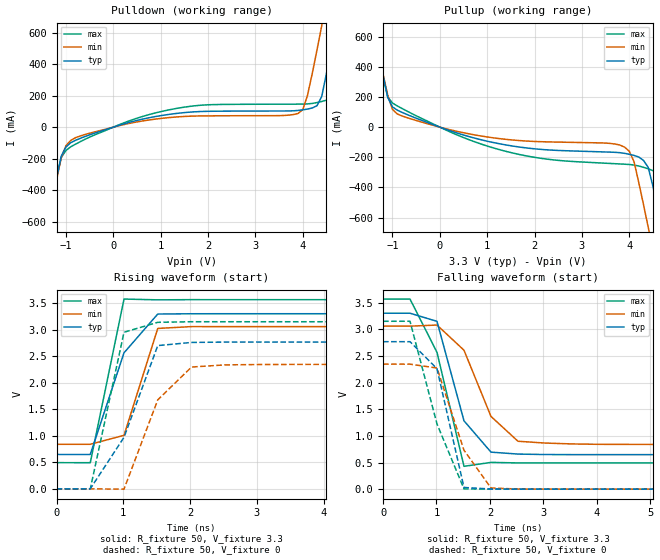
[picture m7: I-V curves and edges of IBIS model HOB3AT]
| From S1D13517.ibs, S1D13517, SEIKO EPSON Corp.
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[Model]   HOB3AT
Model_type Output
Polarity Non-Inverting
C_comp   5p   4p   6p
[Temperature Range] 50   100   0
[Voltage Range]   3.3   3.0   3.6
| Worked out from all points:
|   slope of the pulldown table from 0 to 0.495 V, typ, clamps not added: 11.6 ohm
|   slope of the pullup table from 0 to 0.495 V, typ, clamps not added: 9.57 ohm
|   falling waveform, R_fixture 50, V_fixture 3.3: 20-80 % time 492ps typ, 602ps min, 539ps max; typ from 3.3 V to 0.648 V
|   falling waveform, R_fixture 50, V_fixture 0: 20-80 % time 376ps typ, 562ps min, 586ps max; typ from 2.77 V to 0 V
|   rising waveform, R_fixture 50, V_fixture 3.3: 20-80 % time 508ps typ, 334ps min, 302ps max; typ from 0.648 V to 3.3 V
|   rising waveform, R_fixture 50, V_fixture 0: 20-80 % time 580ps typ, 525ps min, 323ps max; typ from 0 V to 2.77 V
[Pullup]
-3.3V     3.943A     3.608A     4.348A
-1.4V     684.1mA    660.3mA    712.3mA
-1.1V     197.5mA    211.2mA    200.1mA
-800mV    98.34mA    74.29mA    124mA
1.4V      -118.4mA   -81.14mA   -161mA
3.9V      -173.8mA   -132.3mA   -245.9mA
4.1V      -187.6mA   -228.8mA   -251.3mA
4.4V      -266.9mA   -664.2mA   -276.6mA
4.7V      -721.9mA   -1.12A     -342.9mA
4.9V      -1.059A    -1.425A    -612.4mA
5V        -1.228A    -1.577A    -799.5mA
6.6V      -3.945A    -4.028A    -3.853A
[Pulldown]
-3.3V     -3.888A    -3.547A    -4.327A
-1.4V     -659.3mA   -637.4mA   -695.5mA
-1.1V     -183.5mA   -194.3mA   -193.3mA
-1V       -126mA     -116.8mA   -148.1mA
-700mV    -71.52mA   -56.26mA   -92.68mA
1.4V      89.34mA    66.11mA    122.4mA
3.9V      106.1mA    86.91mA    146.2mA
4.1V      114.9mA    202.9mA    147.6mA
4.4V      194.9mA    644.6mA    163.1mA
4.7V      675.1mA    1.105A     215.6mA
5V        1.186A     1.566A     718.4mA
6.6V      3.921A     4.037A     3.78A
[Falling Waveform]
R_fixture=50
V_fixture=3.3
0s        3.3V       3.057V     3.565V
505.1ps   3.3V       3.057V     3.566V
1.01ns    3.148V     3.078V     2.567V
1.515ns   1.282V     2.606V     428.5mV
2.02ns    694.6mV    1.364V     502.2mV
2.525ns   658mV      898.6mV    492.3mV
3.03ns    649.5mV    864.9mV    493.1mV
4.04ns    647.6mV    840.8mV    493mV
5.051ns   647.6mV    838.9mV    492.9mV
50ns      647.6mV    838.8mV    492.9mV
[Falling Waveform]
R_fixture=50
V_fixture=0
0s        2.766V     2.344V     3.149V
505.1ps   2.766V     2.344V     3.149V
1.01ns    2.259V     2.272V     1.223V
1.515ns   31.88mV    730.2mV    4.675mV
2.02ns    2.635mV    23.03mV    803.6uV
2.525ns   682.4uV    2.289mV    177uV
50ns      13.34uV    657.6nV    1.085uV
[Rising Waveform]
R_fixture=50
V_fixture=3.3
0s        647.6mV    838.8mV    492.9mV
505.1ps   647.7mV    838.9mV    491.8mV
1.01ns    2.564V     1.008V     3.576V
1.515ns   3.294V     3.023V     3.562V
2.02ns    3.299V     3.057V     3.565V
50ns      3.3V       3.057V     3.565V
[Rising Waveform]
R_fixture=50
V_fixture=0
0s        0V         0V         0V
505.1ps   11.85uV    -10.88uV   -2.282mV
1.01ns    970.6mV    -6.793mV   2.951V
1.515ns   2.699V     1.677V     3.138V
2.02ns    2.759V     2.295V     3.149V
2.525ns   2.766V     2.336V     3.149V
50ns      2.766V     2.344V     3.149V
[Ramp]
R_load=50
dV/dt_r   1.660E+0/2.427E-10   1.407E+0/3.318E-10   1.889E+0/1.902E-10
dV/dt_f   1.591E+0/4.040E-10   1.355E+0/5.348E-10   1.833E+0/3.078E-10
|[End   HOB3AT
